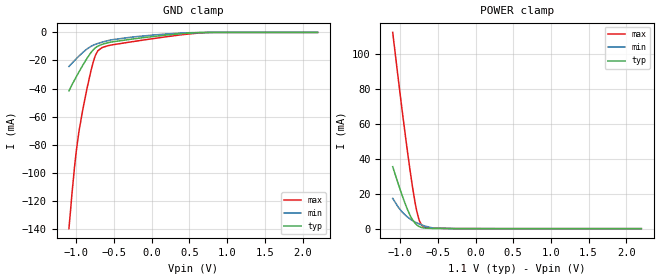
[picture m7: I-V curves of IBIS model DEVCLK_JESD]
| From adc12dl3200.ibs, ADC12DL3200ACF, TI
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|   Model DEVCLK_JESD
[Model]   DEVCLK_JESD
Model_type   Input
Vinl = .57
Vinh = 1.33
|   typ   min   max
|   (nom PVT)   (slow PVT)   (fast PVT)
C_comp   1.800p   1.766p   1.839p
[Voltage Range]   1.1   1.05   1.15
[Temperature Range]   27   125   -40
[Power Clamp Reference]   1.1   1.05   1.15
[GND Clamp Reference]   0   0   0
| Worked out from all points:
|   POWER clamp passes 1 mA (typ) near -0.74 V on its own axis
[GND Clamp]
|   Voltage   I(typ)   I(min)   I(max)
-1.1V     -41.71mA   -24.28mA   -139.9mA
-1.06V    -37.42mA   -22mA      -115.2mA
-1.024V   -33.74mA   -19.96mA   -94.96mA
-1.001V   -31.46mA   -18.69mA   -83.9mA
-964.7mV  -27.95mA   -16.75mA   -69.84mA
-885.5mV  -20.66mA   -12.9mA    -46.68mA
-809.6mV  -14.53mA   -10.03mA   -27.76mA
-760.1mV  -11.49mA   -8.745mA   -18.07mA
-717.2mV  -9.796mA   -7.896mA   -13.12mA
-532.4mV  -6.796mA   -5.272mA   -8.924mA
589.6mV   -251.9uA   -106.3uA   -620.9uA
2.2V      0A         0A         0A
[POWER Clamp]
|   Voltage   I(typ)   I(min)   I(max)
-1.1V     35.42mA    17.32mA    112.2mA
-958.1mV  17.01mA    8.781mA    61.95mA
-908.6mV  11.41mA    6.832mA    45.55mA
-849.2mV  5.951mA    4.947mA    27.24mA
-806.3mV  3.263mA    3.862mA    15.72mA
-779.9mV  2.129mA    3.295mA    9.913mA
-746.9mV  1.169mA    2.667mA    4.702mA
-713.9mV  620.4uA    2.107mA    1.925mA
-667.7mV  293.9uA    1.42mA     638.6uA
-568.7mV  118.7uA    400.3uA    265.1uA
-275mV    18.9uA     5.771uA    73.17uA
2.2V      0A         0A         0A
